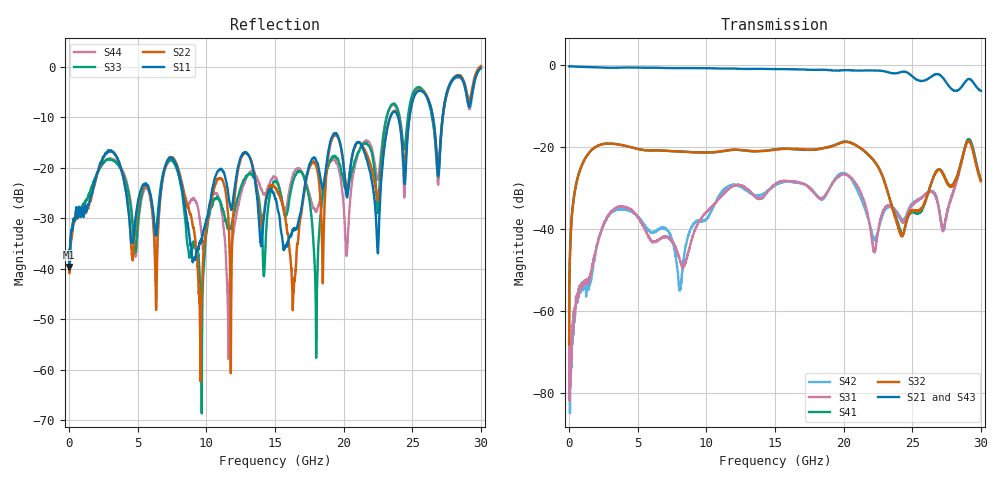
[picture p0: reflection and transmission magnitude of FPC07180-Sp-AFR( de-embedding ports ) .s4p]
!The following data was pulled from an Agilent PNA
!This sNp file was generated from the data in the RF Test software
!NOTE:  Smoothing/Math/Corrections applied on any given trace ARE included in the data saved here
# MHz S dB R 50
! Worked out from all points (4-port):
!   3000 points, 10 MHz to 30 GHz, reference 50 ohm
!   strongest paths, dB at 10 MHz, 7.51 GHz, 15.01 GHz, 22.51 GHz, 30 GHz:
!     S21: -0.2, -0.7, -0.9, -1.2, -6.2
!     S43: -0.2, -0.7, -0.9, -1.3, -6.8
!     S32: -68.1, -20.9, -20.6, -24.7, -28.2
!     S41: -59.2, -20.9, -20.5, -24.8, -27.8
!     S31: -55.7, -42.7, -29.0, -40.6, -27.8
!     S42: -59.7, -42.5, -29.3, -40.5, -27.9
!   lowest |S11| = -39.7 dB at 20 MHz (marker M1), VSWR 1.02, Z = 50.9 + j0.568 ohm
!   |S11| at or under -10 dB: start of sweep to 23.4 GHz; 23.98 GHz to 24.8 GHz (822.8 MHz wide, 3.37 % of centre); 26.51 GHz to 27.21 GHz (701.6 MHz wide, 2.61 % of centre)
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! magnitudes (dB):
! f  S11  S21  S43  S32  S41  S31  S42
! 10 MHz  -36.5  -0.2  -0.2  -68.1  -59.2  -55.7  -59.7
! 20 MHz  -39.7  -0.2  -0.2  -58.3  -58.1  -67.0  -67.2
! 2.33 GHz  -19.1  -0.5  -0.5  -19.3  -19.3  -40.6  -40.5
! 9.57 GHz  -34.7  -0.7  -0.7  -21.2  -21.2  -37.7  -37.9
! 13.17 GHz  -18.0  -0.9  -0.9  -20.8  -20.9  -30.7  -31.1
! 17.99 GHz  -18.5  -1.1  -1.1  -20.5  -20.5  -31.6  -31.5
! 30 GHz  -0.3  -6.2  -6.8  -28.2  -27.8  -27.8  -27.9
